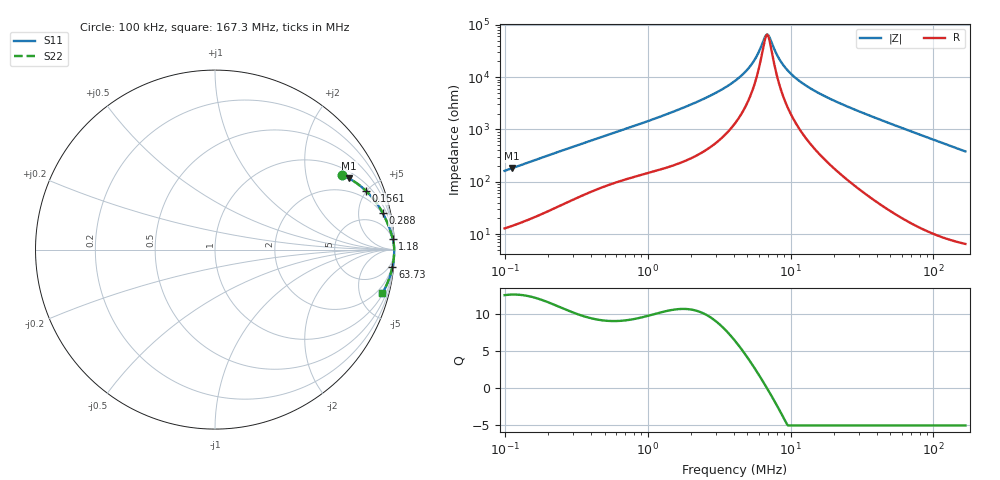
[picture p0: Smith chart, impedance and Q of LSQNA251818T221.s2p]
! LSQNA251818T221  S-PARAMETER MODEL  ( General Type )
! Model Generated by TAIYO YUDEN Corporation (http://www.ty-top.com)
! Version 2.0
! TAIYO YUDEN Control No. 100810NF25SB-FKC
! Copyright(c) 2007 TAIYO YUDEN CO.,LTD. All Rights Reserved.
! Product Description (link to TY-COMPAS)
! https://ds.yuden.co.jp/TYCOMPAS/or/detail?pn=LSQNA251818T221K&u=M
! Products Name : Inductors
! Characteristics :
!  Inductance : 220 uH , SRF(min) : 5.5 MHz , DC Resistance(max) : 5.85 Ohm
!  Rated Current : Saturation :50 mA , Temp Rise : 180 mA (40 degC)
!  Case Size : 2.5 x 1.8 / 0.098 x 0.071 [mm/inch] , Thickness : 1.8 / 0.071 [mm/inch]
!  (Conditions: Temperature = 25 degC , DC Bias Current/Voltage = 0A / 0V)
! External Node Assignments :
!  1  o---GGG---o  2
! GND o---------o GND
! Frequency Range : 0.1MHz  -  167.251077MHz  [ 402 STEP ]
# MHz S RI R 50
! Freq[MHz].  S11 Real  S11 Imag  S21 Real  S21 Imag  S12 Real  S12 Imag  S22 Real  S22 Imag
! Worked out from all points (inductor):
!   401 points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, 100 kHz to 167.3 MHz, reference 50 ohm
!   read as one part in series: L = 254 uH near 103.8 kHz
!   highest Q = 12.7 at 111.8 kHz (marker M1), where L = 256 uH
!   self-resonance near 6.749 MHz
!   S11 on the Smith chart (normalised r, x): 100 kHz: 1.26, +3.22; 156.1 kHz: 1.40, +4.96; 288 kHz: 1.86, +8.90; 1.18 MHz: 4, +34; 63.73 MHz: 1, -20; 167.3 MHz: 1.13, -7.59
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0.1  0.7083 0.4165  0.2917 -0.4165  0.2917 -0.4165  0.7083 0.4165
0.111777  0.7477 0.3966  0.2523 -0.3966  0.2523 -0.3966  0.7477 0.3966
0.1561  0.842 0.3264  0.158 -0.3264  0.158 -0.3264  0.842 0.3264
0.287959  0.9346 0.2036  0.0654 -0.2036  0.0654 -0.2036  0.9346 0.2036
0.346668  0.9494 0.1742  0.0506 -0.1742  0.0506 -0.1742  0.9494 0.1742
1.179696  0.9908 0.058  0.00917 -0.058  0.00917 -0.058  0.9908 0.058
1.20179  0.9911 0.057  0.00892 -0.057  0.00892 -0.057  0.9911 0.057
2.571721  0.9969 0.0244  0.00307 -0.0244  0.00307 -0.0244  0.9969 0.0244
4.166227  0.9981 0.0112  0.00192 -0.0112  0.00192 -0.0112  0.9981 0.0112
5.402077  0.9984 0.00519  0.00165 -0.00519  0.00165 -0.00519  0.9984 0.00519
5.927245  0.9984 0.00315  0.00159 -0.00315  0.00159 -0.00315  0.9984 0.00315
6.625268  0.9985 0.000747  0.00154 -0.000747  0.00154 -0.000747  0.9985 0.000747
6.875753  0.9985 -5.2e-05  0.00153 5.2e-05  0.00153 5.2e-05  0.9985 -5.2e-05
7.135709  0.9985 -0.000852  0.00151 0.000852  0.00151 0.000852  0.9985 -0.000852
8.277601  0.9985 -0.00407  0.00149 0.00407  0.00149 0.00407  0.9985 -0.00407
9.252414  0.9985 -0.00655  0.0015 0.00655  0.0015 0.00655  0.9985 -0.00655
11.13882  0.9984 -0.0109  0.00155 0.0109  0.00155 0.0109  0.9984 -0.0109
14.17747  0.9983 -0.0171  0.00171 0.0171  0.00171 0.0171  0.9983 -0.0171
22.96771  0.9975 -0.0329  0.00251 0.0329  0.00251 0.0329  0.9975 -0.0329
49.14881  0.9927 -0.0753  0.00734 0.0753  0.00734 0.0753  0.9927 -0.0753
63.7281  0.9885 -0.098  0.0115 0.098  0.0115 0.098  0.9885 -0.098
167.2511  0.9315 -0.2441  0.0685 0.2441  0.0685 0.2441  0.9315 -0.2441
